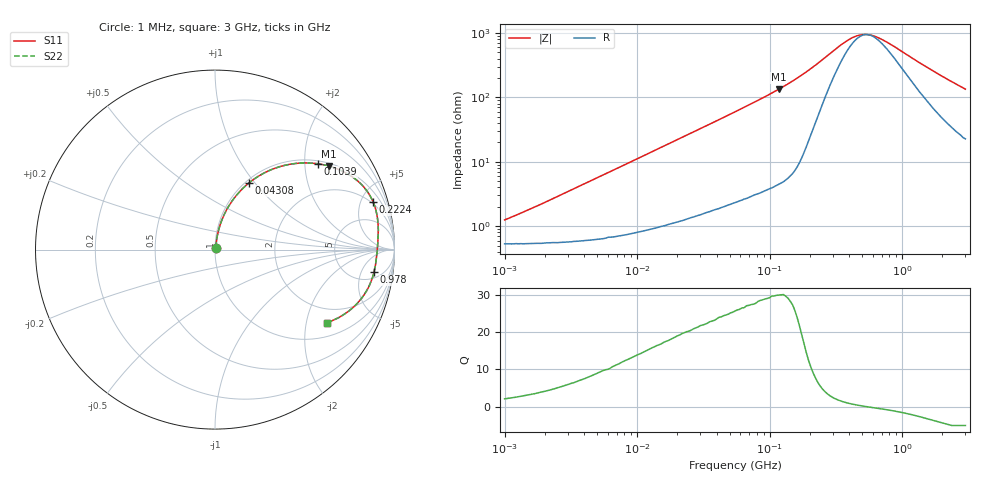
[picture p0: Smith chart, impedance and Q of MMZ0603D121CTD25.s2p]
! S-Parameter Data Generated by TDK Corporation
! Copyright(C) 2025 TDK Corporation.
! All Rights Reserved.
! TDK P/N: MMZ0603D121CTD25 (Chip Bead)
! Property: |Z|=120ohm at 100MHz
! Size(LxWxT): 0.6x0.3x0.3mm
! Model Type: s2p (Touchstone File Format Version 1.0)
! Frequency: DC=Yes Start=1MHz Stop=3000MHz 202points Log-sweep
! Model Generated on Feb. 6, 2025
! Terms and conditions regarding TDK Simulation Models:
! 1)This simulation model is being provided solely for informational
!  purposes. Please refer to the specifications of the products in
!  terms of detailed characteristics of such products.
! 2)In no event shall TDK Corporation of any of its subsidiaries be
!  liable for any loss or damage arising, directly or indirectly,
!  from any information contained in this simulation model, including,
!  but not limited to loss or damages arising from any inaccuracies,
!  omissions or errors in connection with such information.
! 3)Any and all copyrights on this simulation model are owned by
!  TDK Corporation.  Duplication or redistribution of this simulation
!  model without prior written permission from TDK Corporation
!  is prohibited.
! 4)This simulation model is subject to any modification or change
!  without any prior notice.
! 5)Neither TDK Corporation nor any of its subsidiaries shall make any
!  warranty, express or implied, including but not limited to the
!  correctness, implied warranties of merchantability and fitness for
!  a particular purpose with respect to this simulation models.
! 6)The use of this simulation model shall be deemed to have consented
!  to the terms and conditions hereof.
! Port Assignments:
!  1 ---@@@--- 2
! Applicable Conditions:
!  Temperature = 25 degC
!  DC Bias Current = 0 A
!  Small Signal Operation
# Hz S MA R 50
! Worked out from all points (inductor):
!   201 points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, 1 MHz to 3 GHz, reference 50 ohm
!   read as one part in series: L = 180 nH near 1.434 MHz
!   highest Q = 29.9 at 117.2 MHz (marker M1), where L = 181 nH
!   self-resonance near 547 MHz
!   S11 on the Smith chart (normalised r, x): 1 MHz: 1.01, +0.02; 43.08 MHz: 1.04, +0.94; 103.9 MHz: 1.08, +2.33; 222.4 MHz: 1.83, +6.31; 978 MHz: 7, -9; 3 GHz: 1.45, -2.65
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1000000  0.01245 64.2  0.9946 -0.6  0.9946 -0.6  0.01245 64.2
3900413  0.04399 79.8  0.9931 -2.5  0.9931 -2.5  0.04399 79.8
8017732  0.0886 80.3  0.9889 -5.1  0.9889 -5.1  0.0886 80.3
1.461624e7  0.1578 77.5  0.978 -9.1  0.978 -9.1  0.1578 77.5
2.664524e7  0.2759 71.3  0.9481 -16.0  0.9481 -16.0  0.2759 71.3
4.307715e7  0.4174 63.0  0.8916 -24.6  0.8916 -24.6  0.4174 63.0
5.477226e7  0.5032 57.6  0.8448 -30.2  0.8448 -30.2  0.5032 57.6
7.852918e7  0.6418 48.0  0.7441 -39.9  0.7441 -39.9  0.6418 48.0
1.039275e8  0.747 39.8  0.6401 -48.3  0.6401 -48.3  0.747 39.8
1.171891e8  0.7882 36.1  0.5896 -52.0  0.5896 -52.0  0.7882 36.1
1.614254e8  0.8791 26.2  0.4412 -61.4  0.4412 -61.4  0.8791 26.2
2.136344e8  0.9181 17.8  0.3074 -65.8  0.3074 -65.8  0.9181 17.8
2.223601e8  0.9204 16.7  0.2895 -65.9  0.2895 -65.9  0.9204 16.7
3.741707e8  0.9137 5.4  0.1245 -43.5  0.1245 -43.5  0.9137 5.4
4.570858e8  0.908 2.4  0.1004 -22.4  0.1004 -22.4  0.908 2.4
5.154121e8  0.9052 0.8  0.09571 -7.4  0.09571 -7.4  0.9052 0.8
5.81181e8  0.9032 -0.8  0.09763 7.2  0.09763 7.2  0.9032 -0.8
8.005644e8  0.8988 -5.1  0.1314 37.1  0.1314 37.1  0.8988 -5.1
9.779672e8  0.8949 -8.1  0.1696 47.8  0.1696 47.8  0.8949 -8.1
1.347129e9  0.8809 -13.8  0.2545 55.4  0.2545 55.4  0.8809 -13.8
1.782824e9  0.853 -19.7  0.3492 55.6  0.3492 55.6  0.853 -19.7
3e9  0.7438 -33.1  0.5543 47.1  0.5543 47.1  0.7438 -33.1
